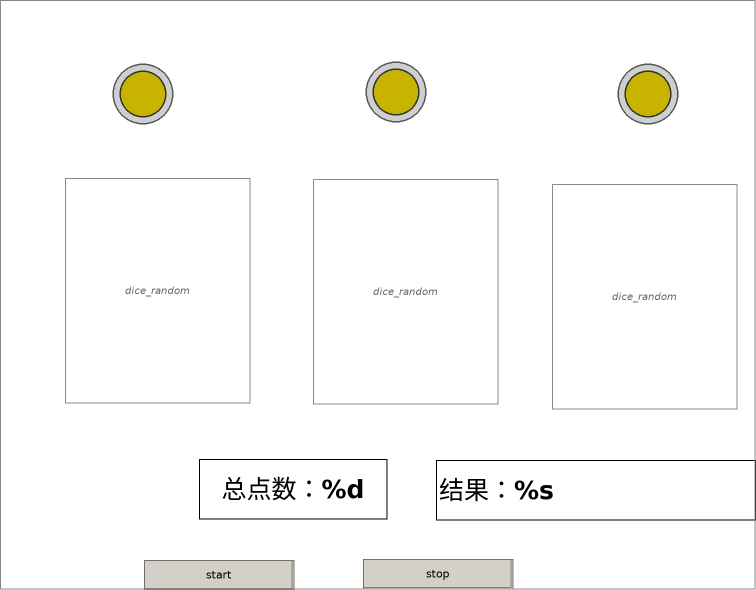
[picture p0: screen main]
VISUALIZATION main  // 756x590
    Button (144,560 150x30), "start"
        tap MAIN.start
    Button (363,559 150x30), "stop"
        tap MAIN.stop
    Frame (65,178 185x225)
        shows dice_random(invisible := MAIN.invisible[1])
    Frame (313,179 185x225)
        shows dice_random(invisible := MAIN.invisible[2])
    Frame (552,184 185x225)
        shows dice_random(invisible := MAIN.invisible[3])
    Rectangle (199,459 188x60), "总点数：%d", text variable: MAIN.totalscore
    Rectangle (436,460 320x60), "结果：%s", text variable: MAIN.stateResult
    Lamp1 (108,59 70x70), variable: MAIN.done[1], style: Lamp-Lamp1-Yellow
    Lamp1 (361,57 70x70), variable: MAIN.done[2], style: Lamp-Lamp1-Yellow
    Lamp1 (613,59 70x70), variable: MAIN.done[3], style: Lamp-Lamp1-Yellow
END_VISUALIZATION
